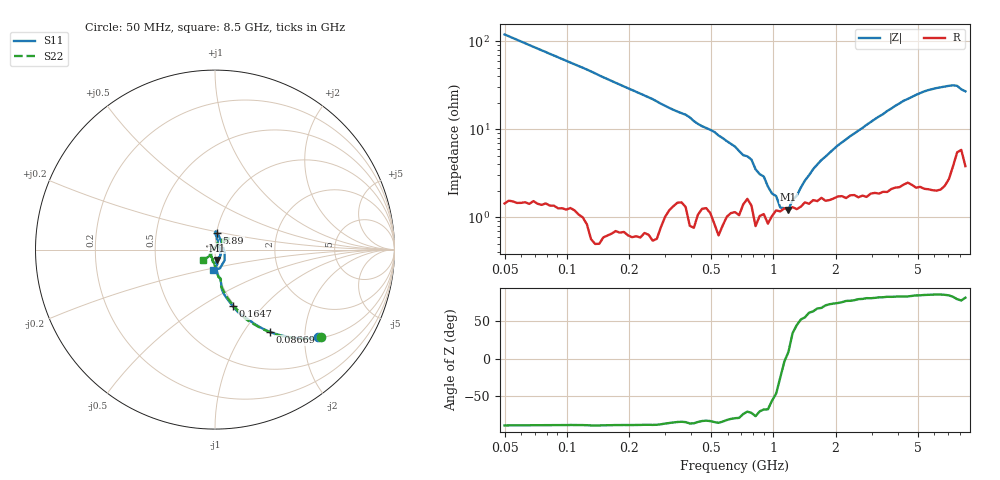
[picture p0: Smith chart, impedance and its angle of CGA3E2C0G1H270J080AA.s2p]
! S-parameter Generated by TDK Corporation
! Copyright(C) 2015 TDK Corporation.
! All Rights Reserved.
! TDK P/N: CGA3E2C0G1H270J080AA (Multilayer Ceramic Chip Capacitors)
! Property: C=27pF
! Size(LxWxT): 1.6x0.8x0.8mm, 0.063x0.031x0.031inches
! Model Type: s2p (Touchstone File Format Version 1.0)
! Frequency: DC=Yes Start=50MHz Stop=8500MHz 114points Log-sweep
! Note:
! Model Generated on Jun. 23, 2015
! Hash(MD5):
! Port Assignments:
!  1 ---| |--- 2
! Applicable Conditions:
!  Temperature = 25 degC
!  DC Bias Voltage = 0 V
!  Small Signal Operation
! Terms and conditions regarding TDK Simulation Models
! (1)This simulation model is being provided solely for informational purposes. Please refer to the specifications of the products in terms of detailed characteristics of such products.
! (2)In no event shall TDK Corporation of any of its subsidiaries be liable for any loss or damage arising, directly or indirectly,
!  From any information contained in this simulation model, including, but not limited to loss or damages arising from any inaccuracies, omissions or errors in connection with such information.
! (3)Any and all copyrights on this simulation model are owned by TDK Corporation.
!  Duplication or redistribution of this simulation model without prior written permission from TDK Corporation is prohibited.
! (4)This simulation model is subject to any modification or change without any prior notice.
! (5)Neither TDK Corporation nor any of its subsidiaries shall make any warranty, express or implied,
!  Including but not limited to the correctness, implied warranties of merchantability and fitness for a particular purpose with respect to this simulation models.
! (6)The use of this simulation model shall be deemed to have consented to the terms and conditions hereof.
# MHz S MA R 50
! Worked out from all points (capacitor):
!   113 points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, 50 MHz to 8.5 GHz, reference 50 ohm
!   read as one part in series: C = 26.7 pF near 50 MHz
!   lowest |Z| = 1.23 ohm at 1.183 GHz (marker M1)
!   series resonance near 1.146 GHz, so ESL is about 720 pH
!   S11 on the Smith chart (normalised r, x): 50 MHz: 1.03, -2.32; 86.69 MHz: 1.01, -1.32; 164.7 MHz: 0.98, -0.69; 5.89 GHz: 1.00, +0.19; 8.5 GHz: 0.95, -0.22
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50  0.753 -40.5  0.6351 49.3  0.6352 49.3  0.7657 -39.7
86.68554  0.5498 -56.4  0.8073 33.7  0.8085 33.8  0.5714 -55.1
119.495  0.4352 -64.2  0.8757 25.9  0.8757 25.9  0.4546 -63.6
164.7224  0.3313 -72.4  0.9249 18.8  0.9249 18.8  0.344 -70.7
285.5811  0.209 -80.0  0.9622 10.1  0.9623 10.1  0.1969 -80.5
651.9202  0.09747 -86.0  0.973 1.6  0.9724 1.7  0.09026 -91.2
1183.275  0.05875 -78.4  0.9749 -3.5  0.974 -3.4  0.05406 -109.7
1558.024  0.0511 -63.5  0.9716 -6.1  0.9721 -6.0  0.0436 -122.3
2354.001  0.03863 -34.0  0.9693 -10.6  0.9684 -10.5  0.03407 -148.5
2701.163  0.03191 -16.3  0.9703 -12.3  0.969 -12.3  0.02467 -160.5
3099.524  0.02873 21.9  0.967 -14.4  0.967 -14.3  0.01252 152.5
3244.963  0.02614 38.1  0.9667 -15.1  0.9663 -15.1  0.01283 107.1
3397.226  0.03112 45.6  0.9672 -15.8  0.9668 -15.9  0.01444 80.9
3723.522  0.04305 67.9  0.9642 -17.6  0.9632 -17.5  0.0352 53.8
4272.658  0.07209 82.4  0.9571 -20.3  0.9576 -20.3  0.0725 43.2
4683.036  0.08497 87.9  0.9562 -22.2  0.9547 -22.1  0.09233 38.2
5889.808  0.09415 83.4  0.9539 -28.3  0.9526 -28.1  0.1039 38.0
7075.547  0.04752 23.8  0.9454 -34.5  0.9458 -34.4  0.05853 62.0
7407.553  0.05573 -14.0  0.9354 -36.2  0.935 -36.3  0.04258 68.4
7755.137  0.08001 -47.8  0.9157 -37.7  0.9162 -37.5  0.01165 74.3
8119.031  0.1082 -75.3  0.9109 -37.9  0.9122 -37.7  0.04127 -128.8
8500  0.1166 -96.7  0.9294 -39.1  0.9327 -38.9  0.08723 -137.6
